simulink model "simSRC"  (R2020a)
settings: Solver=ode15s  StartTime=0.0  StopTime=tsim  FixedStep=tdelay/2  RelTol=1e-3
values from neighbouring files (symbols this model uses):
  d0 = 0    [runSRC.m]    (also in Main.m = [Fh, Tcin, Thin]; Main_OL.m = [Fh, Tcin, Thin]; runTestCalcBlk.m = [Fh, Tcin, Thin]; runTransf.m = [Fh, Tcin, Thin,U0])
  df = 0    [runSRC.m]
  h0 = x0    [runSRC.m]
  hf = h0    [runSRC.m]
  hmax = [2.3; 2.8; 3.2]    [runSRC.m]    (also in TuneSRC.m)
  Kc = Kc*100    [runSRC.m]    (also in TuneSRC.m = double(Kc); Main.m = 1/k*tau/(tauC+theta); runTransf.m = 1/kM(i)*tau(i)/(tauCM(i)+theta(i)); runTransfOL.m = 1/kM(i)*tau(i)/(tauCM(i)+theta(i)))
  nd = length(d0)    [runSRC.m]    (also in Main.m = size(d0,2); Main_OL.m = size(d0,2); runTestCalcBlk.m = size(d0,2); runTransf.m = size(d0,2))
  np = length(param)    [runSRC.m]    (also in runH2Psim.m; Main.m = size(p,2); Main_OL.m = size(p,2); runTestCalcBlk.m = size(p,2))
  nu = length(z0)    [runSRC.m]    (also in runH2Psim.m = length(u0); Main.m = 1; Main_OL.m = 1; runTestCalcBlk.m = 1)
  nx = length(x0)    [runSRC.m]    (also in H2P_Turbine_driven.m = param(end); runTD.m; H2P_Boiler_driven.m = param(end); runBD.m)
  param = [A; Cv; DP; rho; N]    [runSRC.m]    (also in TuneSRC.m = [vmin; vmax; umin; umax; n; price;opening]; runTD.m = [Tref;TrefB;dHvap;cpg;cpW;cpSt;R;Mwt;     T0;TG0;ME;pC;     ; runBD.m = [Tref;TrefB;dHvap;cpg;cpW;cpSt;R;Mwt;          T0;TG0;ME;pC;; runFP.m = [Tref;TrefB;dHvap;cpg;cpW;cpSt;R;Mwt;          T0;TG0;ME;pC;)
  pSR1 = [u01, alpha1, MV]    [runSRC.m]
  pSR2 = [u02, alpha2, MV]    [runSRC.m]
  pSR3 = [u03, alpha3, MV]    [runSRC.m]
  tauI = tauI*1    [runSRC.m]    (also in TuneSRC.m = double(tauI); Main.m = min(tau,4*(tauC+theta)); runTransf.m = min(tau(i), 4*(tauCM(i)+theta(i))); runTransfOL.m = min(tau(i), 4*(tauCM(i)+theta(i))))
  td = 0    [runSRC.m]
  th = ones(6,1)    [runSRC.m]
  tz0OP = [10; tBend]    [runSRC.m]
  tz1OP = [10; tBend]    [runSRC.m]
  tz2OP = [10; tBend]    [runSRC.m]
  tz3OP = [10; tBend]    [runSRC.m]
  v0 = v(end,:)    [runTD.m]    (also in runBD.m; runFP.m; runFPV2.m; runVPC.m)
  x0 = pr/100*hmax    [runSRC.m]    (also in TuneSRC.m = [hH; hH; hH].*hmax; runTD.m = [TE0;TD0;TSh0;MD0; MSh0;w0;TA0;0;0;0;0;0;0;0;0;0]; runBD.m = [TE0;TD0;TSh0;MD0; MSh0;w0;TA0;0;0;0;0;0;0;0;0;0]; runFP.m = [TE0;TD0;TSh0;MD0; MSh0;w0;TA0;0;0;0;0;0;0;0])
  zOP = zOP0-[0.7;0;0;0]    [runSRC.m]
  zOP0 = [1;1;1;1]    [runSRC.m]
undefined symbols (not defined in the file or in its folder): TanksODE

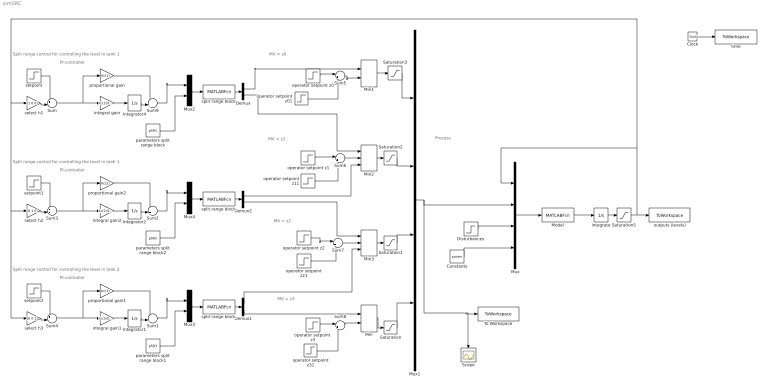
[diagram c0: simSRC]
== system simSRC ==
  note: MV = z3
  note: MV = z2
  note: MV = z1
  note: MV = z0
  note: Process
  note: Split range control for controlling the level in tank 1
  note: PI-controller
  note: PI-controller
  note: Split range control for controlling the level in tank 2
  note: PI-controller
  note: Split range control for controlling the level in tank 1
  Clock : Clock
  Constants : Constant  Value=param
  Demux : Demux  Outputs=2
  Demux1 : Demux  Outputs=2
  Demux2 : Demux  Outputs=2
  Disturbances : Step  Time=td  Before=d0  After=df  SampleTime=0
  Integrator1 : Integrator  InitialCondition=v0(3)
  Integrator2 : Integrator  InitialCondition=v0(2)
  Integrator4 : Integrator  InitialCondition=v0(1)
  Min : MinMax  Inputs=2
  Min1 : MinMax  Inputs=2
  Min2 : MinMax  Inputs=3
  Min3 : MinMax  Inputs=3
  Model : MATLABFcn  MATLABFcn=TanksODE(u(1:nx),u(nx+1:nx+nu),u(nx+nu+1:nx+nu+nd),u(nx+nu+nd+1:nx+nu+nd+np))  OutputDimensions=nx
  Mux : Mux
  Mux1 : Mux
  Mux2 : Mux  Inputs=2
  Mux3 : Mux  Inputs=2
  Mux4 : Mux  Inputs=2
  Saturation{,1..3} (4 alike) : Saturate  UpperLimit=1  LowerLimit=0
  Saturation5 : Saturate  UpperLimit=hmax  LowerLimit=0
  Scope : Scope
  Sum : Sum  Inputs=+-|
  Sum1 : Sum  Inputs=++|
  Sum2 : Sum  Inputs=++|
  Sum3 : Sum  Inputs=+-|
  Sum4 : Sum  Inputs=+-|
  Sum{5..8} (4 alike) : Sum  Inputs=|+-
  Sum9 : Sum  Inputs=++|
  To Workspace : ToWorkspace  VariableName=uSRC  SampleTime=-1
  integral gain : Gain  Gain=Kc(1)/tauI(1)  Multiplication=Matrix(K*u)
  integral gain1 : Gain  Gain=Kc(3)/tauI(3)  Multiplication=Matrix(K*u)
  integral gain2 : Gain  Gain=Kc(2)/tauI(2)  Multiplication=Matrix(K*u)
  integrate : Integrator  InitialCondition=x0
  operator setpoint  z3 : Step  Time=tz3OP(1)  Before=zOP0(4)  After=zOP(4)  SampleTime=0
  operator setpoint z0 : Step  Time=tz0OP(1)  Before=zOP0(1)  After=zOP(1)  SampleTime=0
  operator setpoint z01 : Step  Time=tz0OP(2)  After=zOP(1)-zOP0(1)  SampleTime=0
  operator setpoint z1 : Step  Time=tz1OP(1)  Before=zOP0(2)  After=zOP(2)  SampleTime=0
  operator setpoint z11 : Step  Time=tz1OP(2)  After=zOP(2)-zOP0(2)  SampleTime=0
  operator setpoint z2 : Step  Time=tz2OP(1)  Before=zOP0(3)  After=zOP(3)  SampleTime=0
  operator setpoint z21 : Step  Time=tz2OP(2)  After=zOP(3)-zOP0(3)  SampleTime=0
  operator setpoint z31 : Step  Time=tz3OP(2)  After=zOP(3)-zOP0(3)  SampleTime=0
  outputs (levels) : ToWorkspace  VariableName=ySRC  SampleTime=-1
  parameters split range block : Constant  Value=pSR1
  parameters split range block1 : Constant  Value=pSR3
  parameters split range block2 : Constant  Value=pSR2
  proportional gain : Gain  Gain=Kc(1)  Multiplication=Matrix(K*u)
  proportional gain1 : Gain  Gain=Kc(3)  Multiplication=Matrix(K*u)
  proportional gain2 : Gain  Gain=Kc(2)  Multiplication=Matrix(K*u)
  select h1 : Gain  Gain=[1 0 0]  Multiplication=Matrix(K*u)
  select h2 : Gain  Gain=[0 1 0]  Multiplication=Matrix(K*u)
  select h3 : Gain  Gain=[0 0 1]  Multiplication=Matrix(K*u)
  setpoint : Step  Time=th(1)  Before=h0(1)  After=hf(1)  SampleTime=0
  setpoint1 : Step  Time=th(3)  Before=h0(2)  After=hf(2)  SampleTime=0
  setpoint2 : Step  Time=th(5)  Before=h0(3)  After=hf(3)  SampleTime=0
  "split range block " : MATLABFcn  MATLABFcn=SRblock(u(1),u(2:end))  OutputDimensions=2
  "split range block " : MATLABFcn  MATLABFcn=SRblock(u(1),u(2:end))  OutputDimensions=2
  "split range block " : MATLABFcn  MATLABFcn=SRblock(u(1),u(2:end))  OutputDimensions=2
  time : ToWorkspace  VariableName=tSRC  SampleTime=-1
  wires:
  Clock/1 -> time/1
  Mux/1 -> Model/1
  Model/1 -> integrate/1
  integrate/1 -> Saturation5/1
  Constants/1 -> Mux/4
  Disturbances/1 -> Mux/3
  Mux1/1 -> Scope/1, To Workspace/1, Mux/2
  Saturation3/1 -> Mux1/1
  Saturation2/1 -> Mux1/2
  Saturation1/1 -> Mux1/3
  Saturation/1 -> Mux1/4
  Min/1 -> Saturation/1
  Min2/1 -> Saturation2/1
  Min3/1 -> Saturation1/1
  Min1/1 -> Saturation3/1
  Demux/2 -> Min2/1
  Sum/1 -> proportional gain/1, integral gain/1
  Integrator4/1 -> Sum9/2
  integral gain/1 -> Integrator4/1
  proportional gain/1 -> Sum9/1
  Sum9/1 -> Mux2/1
  Mux2/1 -> "split range block "/1
  parameters split range block/1 -> Mux2/2
  "split range block "/1 -> Demux/1
  Demux/1 -> Min1/1
  Sum1/1 -> Mux3/1
  parameters split range block1/1 -> Mux3/2
  Mux3/1 -> "split range block "/1
  integral gain1/1 -> Integrator1/1
  Integrator1/1 -> Sum1/2
  Demux1/2 -> Min/1
  "split range block "/1 -> Demux1/1
  Sum4/1 -> proportional gain1/1, integral gain1/1
  Demux1/1 -> Min3/3
  proportional gain1/1 -> Sum1/1
  Sum2/1 -> Mux4/1
  parameters split range block2/1 -> Mux4/2
  Mux4/1 -> "split range block "/1
  integral gain2/1 -> Integrator2/1
  Integrator2/1 -> Sum2/2
  Demux2/2 -> Min3/1
  "split range block "/1 -> Demux2/1
  Sum3/1 -> proportional gain2/1, integral gain2/1
  Demux2/1 -> Min2/3
  proportional gain2/1 -> Sum2/1
  Saturation5/1 -> select h3/1, select h2/1, select h1/1, Mux/1, outputs (levels)/1
  select h1/1 -> Sum/2
  setpoint/1 -> Sum/1
  select h2/1 -> Sum3/2
  setpoint1/1 -> Sum3/1
  select h3/1 -> Sum4/2
  setpoint2/1 -> Sum4/1
  operator setpoint z11/1 -> Sum6/2
  operator setpoint z2/1 -> Sum7/1
  operator setpoint z0/1 -> Sum5/1
  operator setpoint  z3/1 -> Sum8/1
  operator setpoint z01/1 -> Sum5/2
  operator setpoint z21/1 -> Sum7/2
  operator setpoint z31/1 -> Sum8/2
  operator setpoint z1/1 -> Sum6/1
  Sum5/1 -> Min1/2
  Sum6/1 -> Min2/2
  Sum7/1 -> Min3/2
  Sum8/1 -> Min/2
